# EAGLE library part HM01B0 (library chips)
ultra low power CMOS Image Sensor 320 x 320
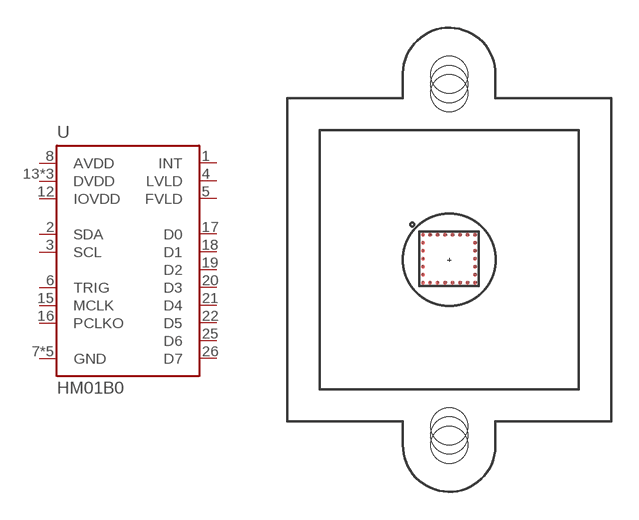
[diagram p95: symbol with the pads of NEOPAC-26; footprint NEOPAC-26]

Designator prefix U

## HM01B0-ANA (MPN: HMB01B0-ANA)  [NEOPAC-26]
1  INT
2  SDA
3  SCL
4  LVLD
5  FVLD
6  TRIG
7  GND
8  AVDD
9  GND
10  GND
11  GND
12  IOVDD
13  DVDD
14  DVDD
15  MCLK
16  PCLKO
17  D0
18  D1
19  D2
20  D3
21  D4
22  D5
23  DVDD
24  GND
25  D6
26  D7

## Footprint NEOPAC-26 (pad centres in mm)
NeoPAC 26 ball grid
smd 0.22 x 0.22: 1 -1.427,1.346; 2 -1.427,0.916; 3 -1.427,0.487; 4 -1.427,0.058; 5 -1.427,-0.371; 6 -1.427,-0.8; 7 -1.427,-1.23; 8 -1.024,-1.23; 9 -0.62,-1.23; 10 -0.217,-1.23; 11 0.187,-1.23; 12 0.591,-1.23; 13 0.994,-1.23; 14 1.398,-1.23; 15 1.398,-0.8; 16 1.398,-0.371; 17 1.398,0.058; 18 1.398,0.487; 19 1.398,0.916; 20 1.398,1.346; 21 0.994,1.346; 22 0.591,1.346; 23 0.187,1.346; 24 -0.217,1.346; 25 -0.62,1.346; 26 -1.024,1.346
hole 2 at 0,10
hole 2 at 0,-10
hole 2 at 0,9
hole 2 at 0,-9
hole 2 at 0,-9.5
hole 2 at 0,9.5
